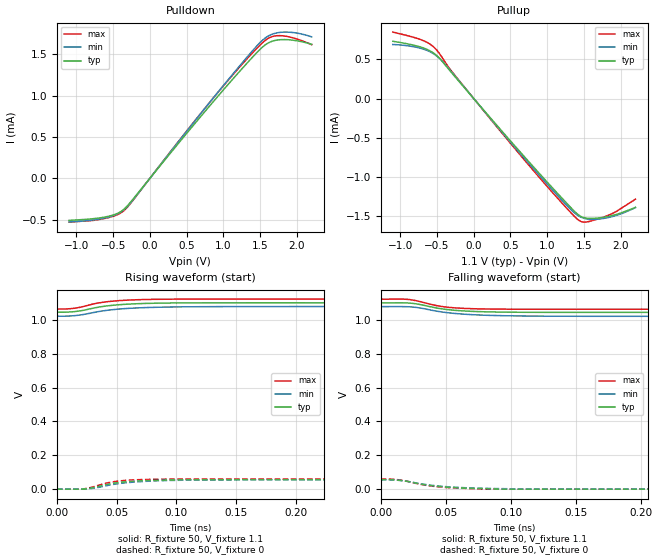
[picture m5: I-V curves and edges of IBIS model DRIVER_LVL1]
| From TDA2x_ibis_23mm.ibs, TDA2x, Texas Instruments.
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| Model based on original model for USB3_PCIEGEN1_PCIEGEN2_TX
|   Sub model DRIVER_LVL1
[model]   DRIVER_LVL1
|[Description]  [1.1V-3-STATE-X-X]
|   , ,
|[Input Load]
|[Output Drive]
|Voltage   1.1V
|Mode   3-STATE
Model_type   3-state
Polarity   Non-Inverting
Enable   Active-Low
Cref =  15.0000pF
Rref =  100.0000M
Vref =  0V
Vmeas =  0.55
C_comp   0   0   0
[Temperature Range]   25   125   -40
[Voltage Range]   1.1   1.078   1.122
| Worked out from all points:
|   slope of the pulldown table from 0 to 0.165 V, typ, clamps not added: 914 ohm
|   slope of the pullup table from 0 to 0.165 V, typ, clamps not added: 916 ohm
|   rising waveform, R_fixture 50, V_fixture 1.1: 20-80 % time 30.6ps typ, 35.6ps min, 27.2ps max; typ from 1.04 V to 1.1 V
|   rising waveform, R_fixture 50, V_fixture 0: 20-80 % time 27.5ps typ, 35.2ps min, 21.9ps max; typ from 0 V to 0.056 V
|   falling waveform, R_fixture 50, V_fixture 1.1: 20-80 % time 27.2ps typ, 33.8ps min, 22.4ps max; typ from 1.1 V to 1.04 V
|   falling waveform, R_fixture 50, V_fixture 0: 20-80 % time 30.8ps typ, 36.3ps min, 27.2ps max; typ from 0.056 V to 0 V
[Pulldown]
-1.1V     -508.8uA   -526.8uA   -530.7uA
-566.7mV  -459.9uA   -469.8uA   -476.3uA
-433.3mV  -421.4uA   -427uA     -436.5uA
-333.3mV  -357.8uA   -364.9uA   -375.5uA
-200mV    -219.6uA   -228.9uA   -231.8uA
900mV     966uA      1.013mA    1.012mA
1.4V      1.469mA    1.546mA    1.521mA
1.567V    1.612mA    1.695mA    1.666mA
1.667V    1.658mA    1.743mA    1.715mA
1.8V      1.677mA    1.767mA    1.723mA
2V        1.662mA    1.756mA    1.684mA
2.2V      1.621mA    1.71mA     1.616mA
[Pullup]
-1.1V     730.9uA    689.9uA    848.6uA
-666.7mV  639.5uA    625.6uA    731.9uA
-566.7mV  593.7uA    583.5uA    676.6uA
-466.7mV  516.1uA    513.3uA    575.6uA
-300mV    329uA      338.6uA    348.6uA
566.7mV   -613.1uA   -630.3uA   -647.4uA
1.2V      -1.273mA   -1.3mA     -1.335mA
1.433V    -1.493mA   -1.504mA   -1.559mA
1.533V    -1.53mA    -1.538mA   -1.578mA
1.767V    -1.518mA   -1.533mA   -1.515mA
1.933V    -1.484mA   -1.496mA   -1.447mA
2.2V      -1.392mA   -1.394mA   -1.286mA
[Ramp]
dV/dt_f 33.832042m/27.441943p 34.486225m/33.842101p 36.101932m/22.776395p
dV/dt_r 33.834669m/27.826301p 33.669785m/35.226966p 36.376843m/22.196849p
R_load = 50
[Rising Waveform]
R_fixture = 50
V_fixture = 1.1
V_fixture_min = 1.078
V_fixture_max = 1.122
0s        1.044V     1.021V     1.063V
9.3ps     1.045V     1.022V     1.064V
14.3ps    1.048V     1.024V     1.067V
21.6ps    1.055V     1.03V      1.077V
34.6ps    1.074V     1.048V     1.099V
48.6ps    1.087V     1.061V     1.111V
67.6ps    1.095V     1.07V      1.118V
94.8ps    1.099V     1.075V     1.121V
207.1ps   1.1V       1.078V     1.122V
1.012ns   1.1V       1.078V     1.122V
[Rising Waveform]
R_fixture = 50
V_fixture = 0
V_fixture_min = 0
V_fixture_max = 0
0s        0V         0V         0V
21.6ps    0V         0V         0V
26.4ps    3.814mV    0V         6.571mV
42.3ps    28.46mV    21.88mV    37.31mV
48.2ps    35.75mV    29.16mV    44.89mV
57.2ps    43.25mV    37.25mV    51.79mV
71.1ps    49.67mV    45.02mV    56.72mV
95.8ps    54.33mV    51.54mV    59.38mV
188.4ps   55.85mV    55.74mV    59.68mV
1.013ns   55.72mV    55.88mV    59.55mV
[Falling Waveform]
R_fixture = 50
V_fixture = 1.1
V_fixture_min = 1.078
V_fixture_max = 1.122
0s        1.1V       1.078V     1.122V
20.3ps    1.1V       1.077V     1.121V
27.7ps    1.094V     1.073V     1.112V
42.6ps    1.07V      1.052V     1.084V
50.9ps    1.061V     1.043V     1.075V
64.7ps    1.052V     1.033V     1.067V
86ps      1.047V     1.026V     1.064V
129.8ps   1.044V     1.022V     1.063V
187.4ps   1.044V     1.021V     1.063V
1.012ns   1.044V     1.021V     1.063V
[Falling Waveform]
R_fixture = 50
V_fixture = 0
V_fixture_min = 0
V_fixture_max = 0
0s        55.72mV    55.88mV    59.55mV
6.8ps     55.72mV    55.88mV    59.55mV
15.1ps    51.72mV    51.29mV    54.17mV
32ps      28.57mV    30.42mV    26.22mV
44.6ps    15.94mV    18.42mV    13.51mV
58.7ps    8.142mV    10.82mV    6.247mV
77.7ps    3.112mV    5.378mV    0V
91.2ps    0V         3.31mV     0V
107.8ps   0V         0V         0V
1.013ns   0V         0V         0V
